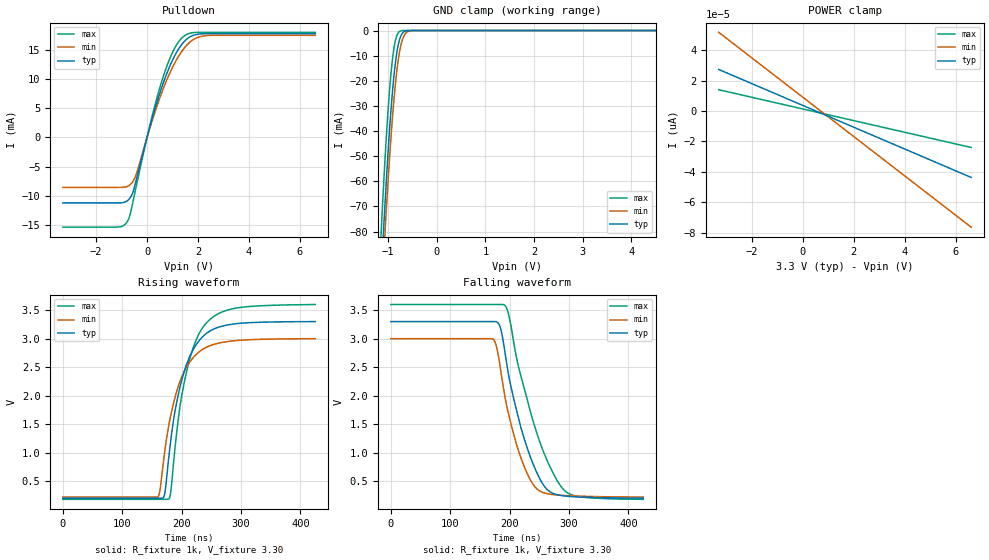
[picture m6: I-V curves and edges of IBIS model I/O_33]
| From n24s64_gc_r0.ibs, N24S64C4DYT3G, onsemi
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|//////////////////////////////////////////////////////////////////////////////
|//////////////////////////////////////////////////////////////////////////////
[Model] I/O_33
Model_type I/O_open_drain
Vinh = 2.31
Vinl = 0.99
Vmeas = 1.65
Vref = 3.30
Rref = 1000
Cref = 100pF
|  variable   typ   min   max
C_comp   8pF   8pF   8pF
|//////////////////////////////////////////////////////////////////////////////
[Temperature Range]   25   85   -40
|//////////////////////////////////////////////////////////////////////////////
[Voltage Range]   3.30V   3.00V   3.60V
|//////////////////////////////////////////////////////////////////////////////
[Pulldown Reference]   0V   0V   0V
|//////////////////////////////////////////////////////////////////////////////
[POWER Clamp Reference] 3.30V   3.00V   3.60V
|//////////////////////////////////////////////////////////////////////////////
[GND Clamp Reference]   0V   0V   0V
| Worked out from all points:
|   slope of the pulldown table from 0 to 0.495 V, typ, clamps not added: 65.7 ohm
|   GND clamp passes 1 mA (typ) near -0.70 V on its own axis
|   falling waveform, R_fixture 1k, V_fixture 3.30: 20-80 % time 45.5ns typ, 38.9ns min, 55.9ns max; typ from 3.3 V to 0.2 V
|   rising waveform, R_fixture 1k, V_fixture 3.30: 20-80 % time 36.1ns typ, 36.7ns min, 35.3ns max; typ from 0.2 V to 3.3 V
|//////////////////////////////////////////////////////////////////////////////
[Pulldown]
|   Voltage   I(typ)   I(min)   I(max)
-3.3V     -11.25mA   -8.58mA    -15.42mA
-1.14V    -11.25mA   -8.58mA    -15.4mA
-780mV    -10.91mA   -8.436mA   -14.52mA
-600mV    -9.907mA   -7.838mA   -12.08mA
-420mV    -7.284mA   -6.304mA   -8.314mA
120mV     1.968mA    1.745mA    2.226mA
540mV     8.138mA    7.273mA    9.13mA
1.02V     13.48mA    12.24mA    14.81mA
1.44V     16.42mA    15.27mA    17.4mA
1.86V     17.63mA    16.95mA    18.06mA
2.34V     17.84mA    17.53mA    18.09mA
6.6V      17.84mA    17.58mA    18.09mA
|//////////////////////////////////////////////////////////////////////////////
[GND Clamp]
|   Voltage   I(typ)   I(min)   I(max)
-3.3V     -907.9mA   -907.8mA   -902.7mA
-1.14V    -97.98mA   -108.6mA   -80.83mA
-1.1V     -83.11mA   -93.77mA   -65.45mA
-1.08V    -76.01mA   -86.92mA   -58.24mA
-1.06V    -68.98mA   -80.12mA   -51.24mA
-940mV    -32.31mA   -43.21mA   -17.68mA
-860mV    -15.12mA   -24.04mA   -5.229mA
-800mV    -6.797mA   -13.46mA   -1.306mA
-740mV    -2.399mA   -6.388mA   -167uA
-640mV    -175uA     -1.159mA   -2.03uA
-500mV    -991.9nA   -23.7uA    -4.902nA
6.6V      27.45pA    55.82pA    12.95pA
|//////////////////////////////////////////////////////////////////////////////
[POWER Clamp]
|   Voltage   I(typ)   I(min)   I(max)
-3.3V     27.45pA    51.92pA    14.1pA
0V        3.732pA    9.127pA    1.413pA
3.3V      -19.99pA   -33.67pA   -11.27pA
6.6V      -43.7pA    -76.47pA   -23.96pA
|//////////////////////////////////////////////////////////////////////////////
|//////////////////////////////////////////////////////////////////////////////
[Ramp]
|  variable   typ   min   max
dV/dt_r   1.860E+00/3.600E-08  1.668E+00/3.600E-08  2.052E+00/3.600E-08
dV/dt_f   1.860E+00/4.500E-08  1.668E+00/3.750E-08  2.052E+00/5.750E-08
R_load = 1k
|//////////////////////////////////////////////////////////////////////////////
|//////////////////////////////////////////////////////////////////////////////
[Falling Waveform]
R_fixture = 1k
V_fixture = 3.30
V_fixture_min = 3.00
V_fixture_max = 3.60
C_fixture = 0p
|   time   V(typ)   V(min)   V(max)
0s        3.3V       3V         3.6V
172.5ns   3.3V       2.991V     3.6V
182.5ns   3.248V     2.615V     3.6V
192.5ns   2.74V      1.963V     3.581V
210ns     1.818V     1.205V     2.754V
237.5ns   856.6mV    474.8mV    1.627V
260ns     389.8mV    287.3mV    938.9mV
285ns     250.6mV    252mV      428.6mV
317.5ns   220.3mV    235.8mV    226.5mV
425ns     200mV      220mV      180mV
|//////////////////////////////////////////////////////////////////////////////
[Rising Waveform]
R_fixture = 1k
V_fixture = 3.30
V_fixture_min = 3.00
V_fixture_max = 3.60
C_fixture = 0p
|   time   V(typ)   V(min)   V(max)
0s        200mV      220mV      180mV
160.5ns   200mV      229.5mV    180mV
171ns     254.6mV    981.3mV    180mV
178.5ns   937.6mV    1.494V     187.6mV
189ns     1.743V     1.977V     1.105V
204ns     2.414V     2.418V     2.212V
219ns     2.801V     2.662V     2.827V
237ns     3.051V     2.823V     3.217V
288ns     3.258V     2.963V     3.53V
425ns     3.3V       3V         3.6V
